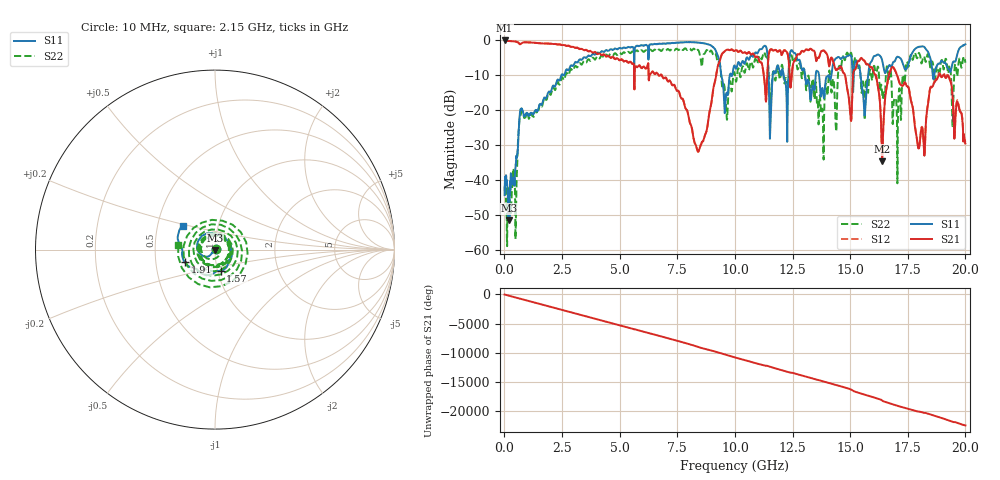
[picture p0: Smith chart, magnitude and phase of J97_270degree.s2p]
!Keysight Technologies,N5222A,MY51421036,A.10.65.16
!Date: Friday, March 31, 2023 14:33:38
!Correction: S11(Full 2 Port(1,2))
!S21(Full 2 Port(1,2))
!S12(Full 2 Port(1,2))
!S22(Full 2 Port(1,2))
!S2P File: Measurements: S11, S21, S12, S22:
# Hz S  dB  R 50
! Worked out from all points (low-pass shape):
!   2000 points, 10 MHz to 20 GHz, reference 50 ohm
!   highest |S21| = -0.02 dB at 10 MHz (marker M1); lowest = -34.6 dB at 16.39 GHz (marker M2)
!   |S21| within 3 dB of the highest: start of sweep to 3.605 GHz; 13.03 GHz to 13.44 GHz (411.1 MHz wide, 3.11 % of centre)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
!   lowest |S11| = -51.5 dB at 200 MHz (marker M3), VSWR 1.01, Z = 50 - j0.267 ohm
!   |S11| at or under -10 dB: start of sweep to 2.472 GHz; 13.05 GHz to 13.51 GHz (461.2 MHz wide, 3.47 % of centre); 13.65 GHz to 14.06 GHz (405 MHz wide, 2.92 % of centre)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
!   |S22| runs from -58.9 to -2.3 dB; largest |S21 - S12| = 0.016
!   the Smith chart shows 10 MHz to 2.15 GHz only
!   S11 on the Smith chart (normalised r, x): 10 MHz: 1.01, +0.01; 1.57 GHz: 1.03, -0.25; 1.91 GHz: 0.71, -0.10; 2.15 GHz: 0.68, +0.19
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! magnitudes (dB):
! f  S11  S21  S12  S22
! 10 MHz  -44.3  0.0  -0.1  -41.8
! 200 MHz  -51.5  -0.2  -0.2  -43.5
! 730 MHz  -19.6  -0.9  -0.8  -20.6
! 1.57 GHz  -18.2  -0.9  -0.8  -18.3
! 1.91 GHz  -14.8  -0.9  -0.9  -15.1
! 2.15 GHz  -13.0  -1.0  -1.0  -13.7
! 3.35 GHz  -5.5  -2.4  -2.4  -7.0
! 6.68 GHz  -1.0  -9.9  -9.8  -2.7
! 8.42 GHz  -0.6  -31.8  -31.8  -2.9
! 9.61 GHz  -15.9  -2.8  -2.8  -18.1
! 10.01 GHz  -7.5  -2.9  -2.9  -10.2
! 13.34 GHz  -14.2  -2.7  -2.7  -12.1
! 13.8 GHz  -13.6  -3.0  -2.9  -20.1
! 14.99 GHz  -4.2  -19.7  -19.7  -4.2
! 15.61 GHz  -20.1  -5.8  -5.7  -17.7
! 15.88 GHz  -6.4  -7.7  -7.6  -8.4
! 16.39 GHz  -5.7  -34.6  -34.6  -15.4
! 16.67 GHz  -7.4  -10.2  -10.1  -11.3
! 17.12 GHz  -4.8  -11.8  -11.7  -14.2
! 17.96 GHz  -1.9  -30.9  -30.7  -3.8
! 19.26 GHz  -8.1  -10.2  -9.9  -9.2
! 20 GHz  -1.1  -29.5  -29.1  -6.4
